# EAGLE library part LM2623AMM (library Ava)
DC/DC Converter
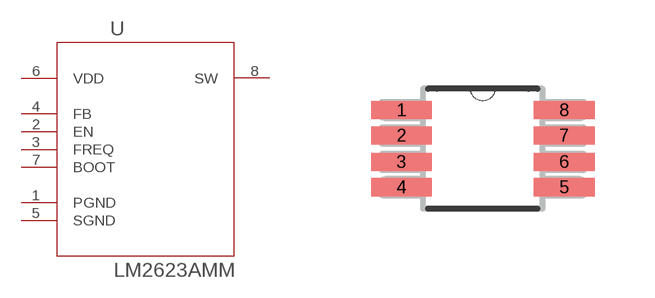
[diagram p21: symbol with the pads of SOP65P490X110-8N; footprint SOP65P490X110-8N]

Designator prefix U

## LM2623AMM (MPN: LM2623AMM; OC_FARNELL: 8207445; OC_NEWARK: 41K3958; PACKAGE: 8-MSOP; SUPPLIER: National Semiconductors)  [SOP65P490X110-8N]
1  PGND  pas
2  EN  in
3  FREQ  in
4  FB  in
5  SGND  pas
6  VDD  pwr
7  BOOT  in
8  SW  out

## Footprint SOP65P490X110-8N (pad centres in mm)
smd 1.524 x 0.457: 1 -2.032,0.965; 2 -2.032,0.33; 3 -2.032,-0.33; 4 -2.032,-0.965; 5 2.032,-0.965; 6 2.032,-0.33; 7 2.032,0.33; 8 2.032,0.965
